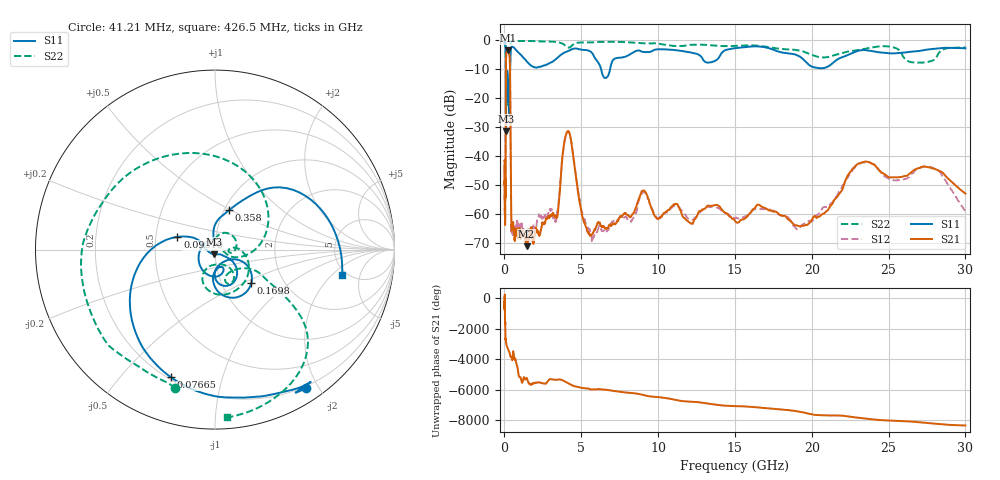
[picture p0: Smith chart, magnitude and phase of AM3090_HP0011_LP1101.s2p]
! Date/Time: Thu, Feb 28, 2019 1:57 PM
! Network Analyzer: Agilent Technologies E8364B Rev: A.07.50.67
! Sweep from 0.010 to 30.000 GHz, 1601 Points, Sweep Type: LOG
! Power Supply: 5.023 V, 0.002 A
# Hz S DB R 50
!freq MagS11 AngS11 MagS21 AngS21 MagS12 AngS12 MagS22 AngS22
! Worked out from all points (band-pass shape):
!   1601 points, 10 MHz to 30 GHz, reference 50 ohm
!   highest |S21| = -3.57 dB at 233.9 MHz (marker M1); lowest = -71.2 dB at 1.439 GHz (marker M2)
!   |S21| within 3 dB of the highest: 103.8 MHz to 343.9 MHz (240.2 MHz wide, 107 % of centre)
!   lowest |S11| = -31.5 dB at 100.9 MHz (marker M3), VSWR 1.05, Z = 49.6 - j2.64 ohm
!   |S11| at or under -10 dB: 91.57 MHz to 369.8 MHz (278.2 MHz wide, 121 % of centre); 6.289 GHz to 6.876 GHz (587.8 MHz wide, 8.93 % of centre)
!   |S22| runs from -31.8 to -0.1 dB; largest |S21 - S12| = 0.013
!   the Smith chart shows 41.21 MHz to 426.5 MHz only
!   S11 on the Smith chart (normalised r, x): 41.21 MHz: 0.17, -1.84; 76.65 MHz: 0.21, -0.69; 93.16 MHz: 0.65, +0.10; 169.8 MHz: 1.37, -0.56; 358 MHz: 1.05, +0.49; 426.5 MHz: 4.59, -2.67
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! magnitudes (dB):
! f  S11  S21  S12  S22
! 10 MHz  -0.3  -41.5  -43.6  -0.7
! 38.04 MHz  -0.5  -60.1  -61.1  -1.7
! 41.21 MHz  -0.7  -59.7  -61.0  -1.9
! 76.65 MHz  -2.5  -45.6  -47.3  -4.4
! 93.16 MHz  -13.1  -14.3  -14.2  -13.4
! 100.9 MHz  -31.5  -7.5  -7.5  -31.4
! 116.1 MHz  -13.7  -4.9  -4.9  -18.8
! 144.7 MHz  -20.4  -3.7  -3.7  -22.1
! 169.8 MHz  -11.2  -3.6  -3.6  -13.5
! 233.9 MHz  -19.9  -3.6  -3.5  -17.5
! 358 MHz  -12.7  -8.7  -8.7  -8.5
! 426.5 MHz  -2.8  -53.8  -54.1  -0.6
! 550.5 MHz  -2.4  -63.9  -66.1  -0.2
! 1.439 GHz  -7.2  -71.2  -67.7  -0.3
! 2.084 GHz  -9.5  -66.1  -64.6  -0.4
! 3.352 GHz  -6.5  -60.8  -62.9  -0.7
! 4.115 GHz  -3.8  -31.5  -31.4  -2.5
! 5.446 GHz  -3.6  -66.2  -64.9  -0.8
! 7.926 GHz  -5.6  -60.1  -61.2  -0.7
! 19.51 GHz  -6.9  -64.1  -63.6  -4.1
! 23.48 GHz  -3.4  -42.0  -42.3  -3.0
! 30 GHz  -2.8  -53.0  -59.1  -2.5
